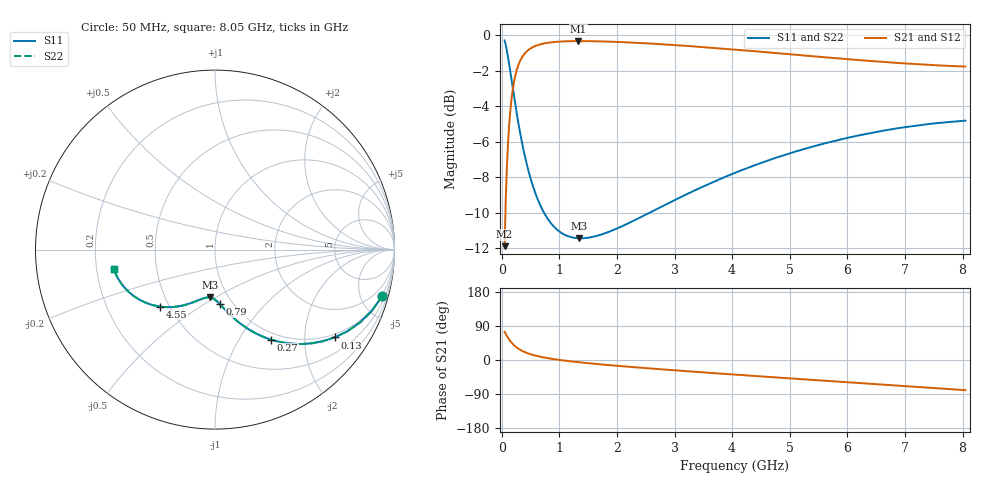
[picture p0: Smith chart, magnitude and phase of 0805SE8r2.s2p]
! AVX Thin Film Operation		Date: August 2001
! Description: Accu-P® Series, Thin Film, SMD, RF Capacitor
! Part Number: 08051J8R2BBT
! 50 MHz  -  8.05 GHz
! Serial Measurements
# mhz S db R 50
!	S11		S21		S12		S22
!	dB	Phase	dB	Phase	dB	Phase	dB	Phase
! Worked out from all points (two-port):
!   401 points, 50 MHz to 8.05 GHz, reference 50 ohm
!   highest |S21| = -0.33 dB at 1.33 GHz (marker M1); lowest = -11.9 dB at 50 MHz (marker M2)
!   |S21| within 3 dB of the highest: 180.6 MHz to end of sweep
!   lowest |S11| = -11.4 dB at 1.35 GHz (marker M3), VSWR 1.73, Z = 41.2 - j23.6 ohm
!   |S11| at or under -10 dB: 733.8 MHz to 2.568 GHz (1.834 GHz wide, 111 % of centre)
!   |S22| runs from -11.4 to -0.3 dB; largest |S21 - S12| = 0
!   S11 on the Smith chart (normalised r, x): 50 MHz: 0.90, -7.22; 130 MHz: 0.90, -2.79; 270 MHz: 0.90, -1.38; 790 MHz: 0.87, -0.59; 4.55 GHz: 0.45, -0.35; 8.05 GHz: 0.27, -0.09
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50  -0.29 -15.5  -11.89 74.5  -11.89 74.5  -0.29 -15.5
90  -0.88 -26.7  -7.40 63.3  -7.40 63.3  -0.88 -26.7
110  -1.25 -31.7  -6.04 58.3  -6.04 58.3  -1.25 -31.7
130  -1.65 -36.2  -5.01 53.7  -5.01 53.7  -1.65 -36.3
190  -2.93 -47.5  -3.09 42.5  -3.09 42.5  -2.93 -47.5
230  -3.78 -53.4  -2.36 36.6  -2.36 36.6  -3.78 -53.4
270  -4.59 -58.2  -1.86 31.8  -1.86 31.8  -4.59 -58.2
350  -6.02 -65.6  -1.25 24.4  -1.25 24.4  -6.02 -65.6
470  -7.71 -73.2  -0.81 16.8  -0.81 16.8  -7.71 -73.2
610  -9.13 -79.3  -0.57 10.7  -0.57 10.7  -9.13 -79.3
790  -10.30 -84.8  -0.43 5.1  -0.43 5.1  -10.30 -84.9
1030  -11.13 -90.3  -0.35 -0.4  -0.35 -0.4  -11.13 -90.3
1330  -11.44 -95.7  -0.33 -5.8  -0.33 -5.8  -11.44 -95.7
1350  -11.44 -96.0  -0.33 -6.1  -0.33 -6.1  -11.44 -96.0
1390  -11.44 -96.6  -0.33 -6.7  -0.33 -6.7  -11.44 -96.6
1990  -10.91 -105.0  -0.37 -15.1  -0.37 -15.1  -10.91 -105.1
2730  -9.73 -114.0  -0.49 -24.1  -0.49 -24.1  -9.73 -114.0
4050  -7.75 -128.5  -0.81 -38.6  -0.81 -38.6  -7.75 -128.5
4550  -7.14 -133.7  -0.94 -43.8  -0.94 -43.8  -7.14 -133.7
5390  -6.28 -142.3  -1.18 -52.4  -1.18 -52.4  -6.28 -142.3
6730  -5.32 -155.9  -1.53 -66.0  -1.53 -66.0  -5.32 -155.9
8050  -4.82 -169.4  -1.76 -79.6  -1.76 -79.6  -4.82 -169.4
